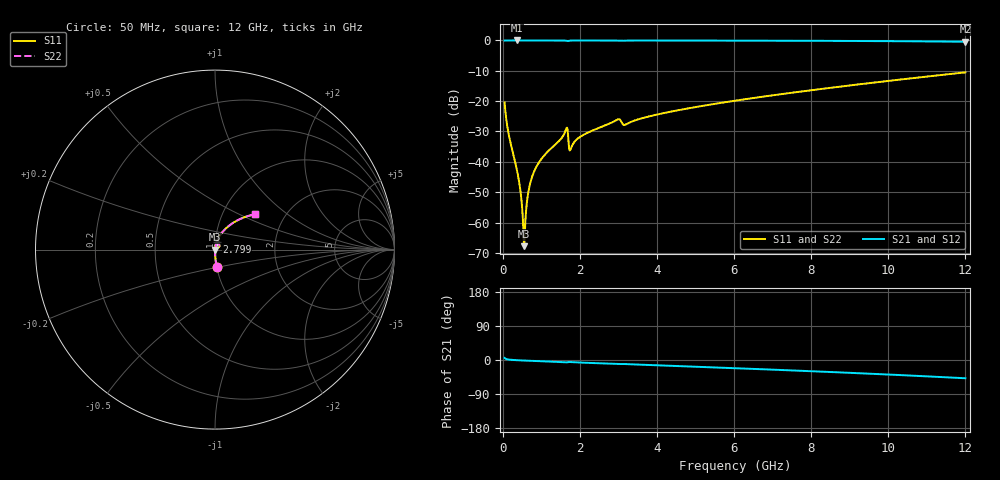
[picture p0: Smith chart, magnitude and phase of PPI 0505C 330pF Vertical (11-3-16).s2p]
# GHz S MA R 50
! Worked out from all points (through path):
!   1601 points, 50 MHz to 12 GHz, reference 50 ohm
!   highest |S21| = 0.00 dB at 363.7 MHz (marker M1); lowest = -0.4 dB at 12 GHz (marker M2)
!   group delay of S21, straight-line fit = 11.1 ps
!   lowest |S11| = -67.8 dB at 557.9 MHz (marker M3), VSWR 1.00, Z = 50 + j0.0039 ohm
!   |S11| at or under -10 dB: start of sweep to end of sweep
!   |S22| runs from -67.8 to -10.5 dB; largest |S21 - S12| = 0
!   S11 on the Smith chart (normalised r, x): 50 MHz: 1.00, -0.19; 2.799 GHz: 1.01, +0.09; 12 GHz: 1.42, +0.61
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0.05  0.09514 -84.6  0.9953 5.3  0.9953 5.3  0.09514 -84.6
0.1695  0.02579 -88.4  0.9994 1.0  0.9994 1.0  0.02579 -88.4
0.3636875  0.007612 -87.9  0.9996 -0.5  0.9996 -0.5  0.007612 -87.9
0.4458437  0.003899 -85.5  0.9996 -1.0  0.9996 -1.0  0.003899 -85.5
0.5205313  0.001224 -72.5  0.9996 -1.3  0.9996 -1.3  0.001224 -72.5
0.557875  0.0004075 5.5  0.9996 -1.5  0.9996 -1.5  0.0004075 5.5
0.5952188  0.001252 69.0  0.9995 -1.6  0.9995 -1.6  0.001252 69.0
0.6549687  0.0029 79.6  0.9995 -1.9  0.9995 -1.9  0.0029 79.6
0.7221875  0.004648 82.3  0.9995 -2.2  0.9995 -2.2  0.004648 82.3
0.8192812  0.007002 83.6  0.9995 -2.6  0.9995 -2.6  0.007002 83.6
0.9537187  0.01005 84.0  0.9994 -3.1  0.9994 -3.1  0.01005 84.0
1.625906  0.03208 73.2  0.9934 -6.1  0.9934 -6.1  0.03208 73.2
1.775281  0.01694 70.9  0.9958 -5.6  0.9958 -5.6  0.01694 70.9
2.044156  0.02666 80.9  0.9985 -6.9  0.9985 -6.9  0.02666 80.9
2.7985  0.0434 77.9  0.9972 -9.9  0.9972 -9.9  0.0434 77.9
3.000156  0.05041 70.3  0.9907 -10.8  0.9907 -10.8  0.05041 70.3
3.179406  0.04083 71.0  0.9931 -10.7  0.9931 -10.7  0.04083 71.0
4.038312  0.0608 74.9  0.9968 -14.1  0.9968 -14.1  0.0608 74.9
6.025  0.1016 67.7  0.9933 -21.6  0.9933 -21.6  0.1016 67.7
8.019156  0.1518 59.9  0.9865 -29.6  0.9865 -29.6  0.1518 59.9
10.01331  0.2159 51.2  0.9741 -38.4  0.9741 -38.4  0.2159 51.2
12  0.2978 41.4  0.9517 -48.2  0.9517 -48.2  0.2978 41.4
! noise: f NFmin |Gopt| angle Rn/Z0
0.05  0.0003103  0.8329  0.224  0.0003918
1.372  0.003257  0.6151  3.488  0.001572
2.701  0.005955  0.592  6.79  0.002666
4.031  0.006962  0.5078  9.766  0.002439
5.36  0.0082  0.4626  12.48  0.002543
6.682  0.009738  0.445  15.12  0.002876
8.012  0.0114  0.4377  17.66  0.00329
9.341  0.01322  0.4379  20.13  0.003791
10.67  0.01522  0.4445  22.55  0.004408
12  0.01749  0.457  24.97  0.005187
